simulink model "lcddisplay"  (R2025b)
settings: Solver=FixedStepAuto  StartTime=0.0  StopTime=10.0  RelTol=1e-3  EnableMultiTasking=on
libraries: simulink x1

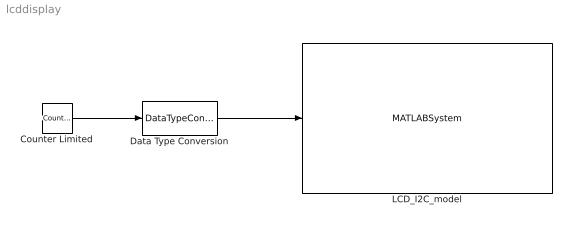
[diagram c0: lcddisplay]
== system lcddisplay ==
  Counter Limited : simulink/Sources/Counter Limited  uplimit=255  tsamp=-1
  Data Type Conversion : DataTypeConversion  OutDataTypeStr=int8
  LCD_I2C_model : MATLABSystem  System=LCD_I2C  SampleTime=-1
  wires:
  Counter Limited/1 -> Data Type Conversion/1
  Data Type Conversion/1 -> LCD_I2C_model/1
